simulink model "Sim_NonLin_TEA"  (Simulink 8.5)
settings: Solver=ode45  StartTime=0.0  StopTime=25*3600  RelTol=1e-3
InitFcn:
  | start
StopFcn:
  | pl2
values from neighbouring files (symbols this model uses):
  ini = [wbo; atto; Hco]    [start.m]    (also in start1.m; start2.m; start3.m)
  Kpqr = lqr(sys,Q0,R0)    [des.m]
  nt = 12    [start.m]    (also in start1.m; start2.m; start3.m)
  r2d = 180/pi    (= 57.2957795131)    [start.m]    (also in start1.m; start2.m; start3.m)
  wo = 0.0011    [start.m]    (also in start1.m; start2.m; start3.m)
undefined symbols (not defined in the file or in its folder): Rigbod_Dynam_LVLH

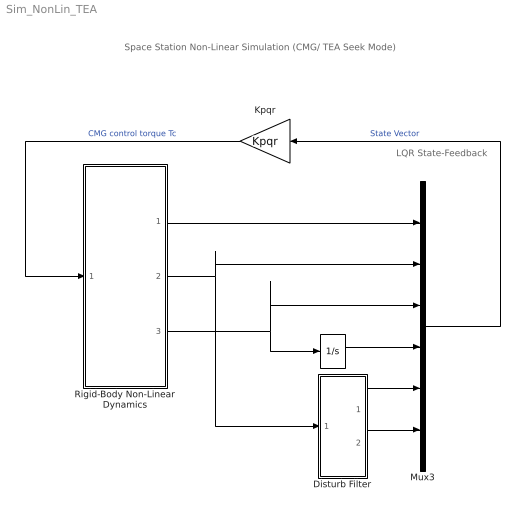
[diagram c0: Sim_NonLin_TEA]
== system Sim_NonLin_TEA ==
  note: Space Station Non-Linear Simulation (CMG/ TEA Seek Mode)
  note: LQR State-Feedback
  "  " : Integrator
  Disturb Filter : Subsystem
  Kpqr : Gain  Gain=Kpqr  Multiplication=Matrix(K*u)
  Mux3 : Mux  Inputs=[3, 3, 3, 3, 1, 1]
  Rigid-Body Non-Linear Dynamics : Subsystem
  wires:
  "  "/1 -> Mux3/4
  Kpqr/1 -> Rigid-Body Non-Linear Dynamics/1(Tcmg)  "CMG control torque Tc"
  Mux3/1 -> Kpqr/1  "State Vector"
  Disturb Filter/1(a1) -> Mux3/5
  Disturb Filter/2(a2) -> Mux3/6
  Rigid-Body Non-Linear Dynamics/3(Hcmg) -> "  "/1, Mux3/3
  Rigid-Body Non-Linear Dynamics/2(att) -> Disturb Filter/1(the), Mux3/2
  Rigid-Body Non-Linear Dynamics/1(Wl) -> Mux3/1

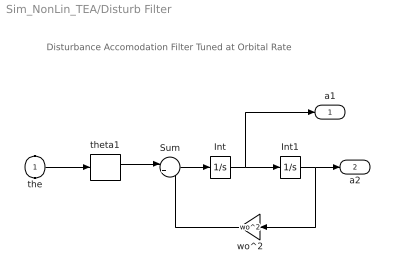
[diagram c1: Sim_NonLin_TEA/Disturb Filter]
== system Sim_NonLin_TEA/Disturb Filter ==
  note: Disturbance Accomodation Filter Tuned at Orbital Rate
  the : Inport
  Int : Integrator
  Int1 : Integrator
  Sum : Sum  Inputs=|+-
  theta1 : Selector  InputPortWidth=3  Indices=[2]
  wo^2 : Gain  Gain=wo^2
  a1 : Outport
  a2 : Outport  Port=2
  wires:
  Int/1 -> Int1/1, a1/1
  Sum/1 -> Int/1
  Int1/1 -> wo^2/1, a2/1
  wo^2/1 -> Sum/2
  theta1/1 -> Sum/1
  the/1 -> theta1/1

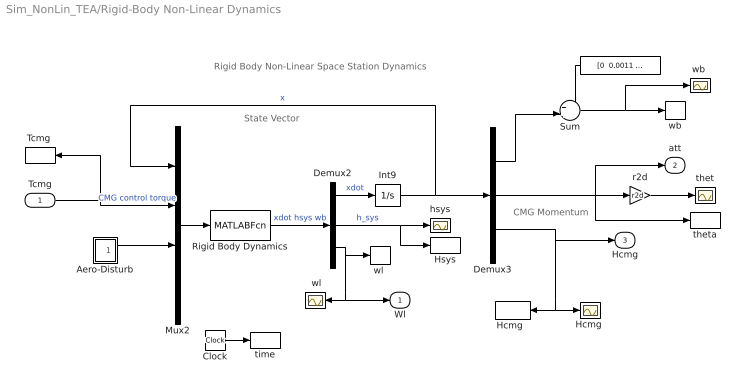
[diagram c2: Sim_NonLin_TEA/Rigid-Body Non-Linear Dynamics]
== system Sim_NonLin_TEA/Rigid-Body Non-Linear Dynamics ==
  note: Rigid Body Non-Linear Space Station Dynamics
  note: State Vector
  note: CMG Momentum
  Tcmg : Inport  PortDimensions=3
  " " : Constant  Value="[0  0.0011  0]"
  " wl" : Scope
  Aero-Disturb : Subsystem
  Clock : Clock
  Demux2 : Demux  Outputs=[9,3,3]
  Demux3 : Demux  Outputs=[3,3,3]
  "Hcmg " : Scope
  "Hcmg  " : ToWorkspace  VariableName=Hcmg  SampleTime=-1
  Hsys : ToWorkspace  VariableName=Hsys  SampleTime=-1
  Int9 : Integrator  InitialCondition=ini
  Mux2 : Mux  Inputs=[9, 3, 3, nt]
  Rigid Body Dynamics : MATLABFcn  MATLABFcn=Rigbod_Dynam_LVLH( u(1:9), u(10:12), u(13:15), u(16:15+nt) )  OutputDimensions=15
  Sum : Sum  Inputs=++|
  "Tcmg " : ToWorkspace  VariableName=Tcmg  SampleTime=-1
  hsys : Scope
  r2d : Gain  Gain=r2d
  thet : Scope
  theta : ToWorkspace  VariableName=theta  SampleTime=-1
  time : ToWorkspace  VariableName=time  SampleTime=-1
  wb : ToWorkspace  VariableName=wb  SampleTime=-1
  "wb " : Scope
  "wl " : ToWorkspace  VariableName=wl  SampleTime=-1
  Wl : Outport
  att : Outport  Port=2
  Hcmg : Outport  Port=3
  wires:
  Rigid Body Dynamics/1 -> Demux2/1  "xdot hsys wb"
  Demux2/1 -> Int9/1  "xdot"
  Int9/1 -> Demux3/1, Mux2/1  "x"
  Tcmg/1 -> Mux2/2, "Tcmg "/1  "CMG control torque"
  Demux2/3 -> "wl "/1, " wl"/1, Wl/1
  Demux2/2 -> hsys/1, Hsys/1  "h_sys"
  Demux3/2 -> r2d/1, theta/1, att/1
  Demux3/3 -> "Hcmg  "/1, "Hcmg "/1, Hcmg/1
  r2d/1 -> thet/1
  Clock/1 -> time/1
  Mux2/1 -> Rigid Body Dynamics/1
  Sum/1 -> "wb "/1, wb/1
  Demux3/1 -> Sum/2
  " "/1 -> Sum/1
  Aero-Disturb/1(Td) -> Mux2/3

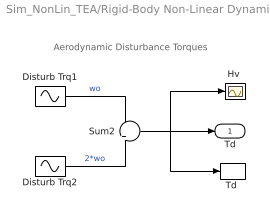
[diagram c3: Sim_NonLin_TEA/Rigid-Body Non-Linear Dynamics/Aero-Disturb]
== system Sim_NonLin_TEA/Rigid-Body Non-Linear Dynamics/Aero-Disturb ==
  note: Aerodynamic Disturbance Torques
  Disturb Trq1 : Sin  Amplitude=[1, 3, 1]  Bias="[1  8  1]"  Frequency=[wo, wo, wo]  SampleTime=0
  Disturb Trq2 : Sin  Amplitude=[1, 1, 1]*0.5  Frequency=[wo, wo, wo]*2  SampleTime=0
  "Hv " : Scope
  Sum2 : Sum  Inputs=+|+
  "Td " : ToWorkspace  VariableName=Td  SampleTime=-1
  Td : Outport
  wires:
  Disturb Trq1/1 -> Sum2/1  "wo"
  Sum2/1 -> "Td "/1, "Hv "/1, Td/1
  Disturb Trq2/1 -> Sum2/2  "2*wo"
